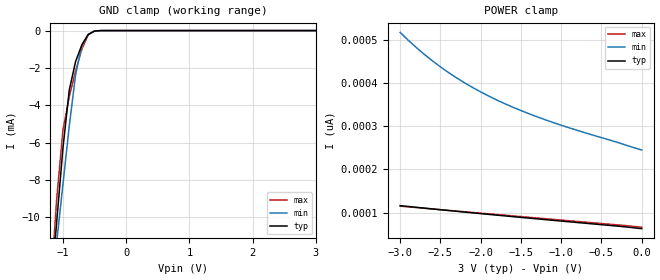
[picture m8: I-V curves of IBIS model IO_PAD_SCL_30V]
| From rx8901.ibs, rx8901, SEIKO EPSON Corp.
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[Model]   IO_PAD_SCL_30V
Model_type Input
Polarity Non-Inverting
Vinh=2.10
Vinl=0.90
C_comp   2.5p   2.0p   3.0p
[Temperature Range] 25   105   -40
[Voltage Range]   3.00   2.70   3.30
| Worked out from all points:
|   GND clamp passes 1 mA (typ) near -0.73 V on its own axis
[GND Clamp]
-3V       -89.09mA   -73.03mA   -108.2mA
-1.2V     -14.35mA   -14.54mA   -14.15mA
-1.1V     -10.3mA    -11.38mA   -9.07mA
-1V       -6.3mA     -8.234mA   -5.326mA
-900mV    -3.191mA   -5.116mA   -3.551mA
-800mV    -1.656mA   -2.369mA   -2.158mA
-700mV    -763.9uA   -781.8uA   -983.1uA
-600mV    -207.7uA   -205.1uA   -228.8uA
-500mV    -21.87uA   -34.9uA    -13.49uA
-300mV    -47nA      -341.4nA   -3.543nA
3V        62.76pA    262.6pA    59.86pA
[POWER Clamp]
-3V       116pA      517.4pA    114.8pA
-2.9V     114.1pA    499.3pA    113.2pA
-2.7V     110.3pA    466.4pA    110pA
-2.6V     108.4pA    451.5pA    108.4pA
-2.4V     104.8pA    424.4pA    105.2pA
-2.1V     99.36pA    389.7pA    100.4pA
-1.8V     94.08pA    360.8pA    95.56pA
-1.5V     88.88pA    336.3pA    90.75pA
-1.1V     82.06pA    308.7pA    84.35pA
0V        62.76pA    244.9pA    66.01pA
